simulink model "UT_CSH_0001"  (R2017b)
settings: Solver=FixedStepDiscrete  StartTime=0.0  StopTime=2  FixedStep=0.01  RelTol=1e-3  EnableMultiTasking=on
undefined symbols (not defined in the file): sigbuilder_block

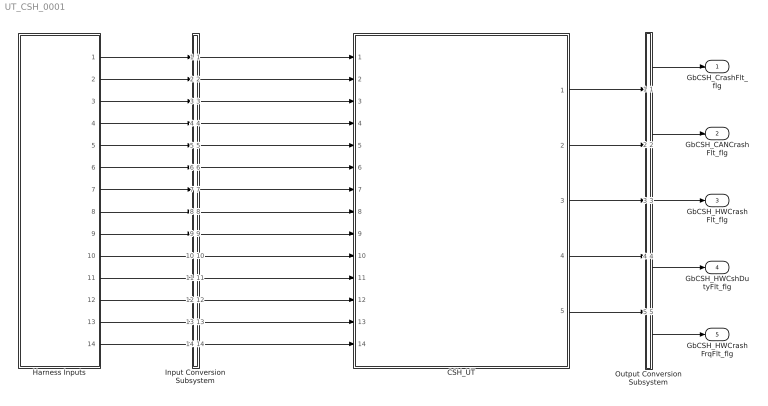
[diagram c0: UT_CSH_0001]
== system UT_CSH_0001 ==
  CSH_UT : ModelReference  ModelNameDialog=CSH_UT  SimulationMode=Normal  ModelReferenceVersion='M102C102'
  Harness Inputs : Subsystem  Tag=STV Subsys  LoadFcn=sigbuilder_block('load');  StartFcn=sigbuilder_block('start');  StopFcn=sigbuilder_block('stop');  ClipboardFcn=sigbuilder_block('clipboard');  mask(Sigbuilder block){tuvar=[0:10]}
      mask init:
      | if ~strcmp(get_param(bdroot(gcb),'SimulationStatus'),'stopped'),tuvar = sigbuilder_block('maskInit'); end
  Input Conversion Subsystem : Subsystem  Tag=__SLT_ICS__  Description=Signal spec. and routing
  Output Conversion Subsystem : Subsystem  Tag=__SLT_OCS__  Description=Signal spec. and routing
  GbCSH_CrashFlt_flg : Outport  OutDataTypeStr=boolean  PortDimensions=[1]
  GbCSH_CANCrashFlt_flg : Outport  Port=2  OutDataTypeStr=boolean  PortDimensions=[1]
  GbCSH_HWCrashFlt_flg : Outport  Port=3  OutDataTypeStr=boolean  PortDimensions=[1]
  GbCSH_HWCshDutyFlt_flg : Outport  Port=4  OutDataTypeStr=boolean  PortDimensions=[1]
  GbCSH_HWCrashFrqFlt_flg : Outport  Port=5  OutDataTypeStr=boolean  PortDimensions=[1]
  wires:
  Harness Inputs/1(GeADP_CrashSgl_enum) -> Input Conversion Subsystem/1(Inport_1)
  Harness Inputs/2(GcLDP_CshDutyOut_pct) -> Input Conversion Subsystem/2(Inport_2)
  Harness Inputs/3(GcLDP_CshPerOut_ms) -> Input Conversion Subsystem/3(Inport_3)
  Harness Inputs/4(GcLDP_CshSt_numb) -> Input Conversion Subsystem/4(Inport_4)
  Harness Inputs/5(GcLDP_CshDutyFbk_pct) -> Input Conversion Subsystem/5(Inport_5)
  Harness Inputs/6(GcLDP_CshPerFbk_ms) -> Input Conversion Subsystem/6(Inport_6)
  Harness Inputs/7(GcLDP_CshStFbk_numb) -> Input Conversion Subsystem/7(Inport_7)
  Harness Inputs/8(GbWSM_Kl15WkUpPrs_flg) -> Input Conversion Subsystem/8(Inport_8)
  Harness Inputs/9(GbUDS_TestMode1_flg) -> Input Conversion Subsystem/9(Inport_9)
  Harness Inputs/10(GeUDS_PrjSel_enum) -> Input Conversion Subsystem/10(Inport_10)
  Harness Inputs/11(GbADP_050ChkSum_flg) -> Input Conversion Subsystem/11(Inport_11)
  Harness Inputs/12(GbADP_050RCMsg_flg) -> Input Conversion Subsystem/12(Inport_12)
  Harness Inputs/13(GbISP_TF050ChkSum_flg) -> Input Conversion Subsystem/13(Inport_13)
  Harness Inputs/14(GbISP_TF050RCMsg_flg) -> Input Conversion Subsystem/14(Inport_14)
  Output Conversion Subsystem/1(Outport_1) -> GbCSH_CrashFlt_flg/1
  Output Conversion Subsystem/2(Outport_2) -> GbCSH_CANCrashFlt_flg/1
  Output Conversion Subsystem/3(Outport_3) -> GbCSH_HWCrashFlt_flg/1
  Output Conversion Subsystem/4(Outport_4) -> GbCSH_HWCshDutyFlt_flg/1
  Output Conversion Subsystem/5(Outport_5) -> GbCSH_HWCrashFrqFlt_flg/1
  Input Conversion Subsystem/1(Outport_1) -> CSH_UT/1
  Input Conversion Subsystem/2(Outport_2) -> CSH_UT/2
  Input Conversion Subsystem/3(Outport_3) -> CSH_UT/3
  Input Conversion Subsystem/4(Outport_4) -> CSH_UT/4
  Input Conversion Subsystem/5(Outport_5) -> CSH_UT/5
  Input Conversion Subsystem/6(Outport_6) -> CSH_UT/6
  Input Conversion Subsystem/7(Outport_7) -> CSH_UT/7
  Input Conversion Subsystem/8(Outport_8) -> CSH_UT/8
  Input Conversion Subsystem/9(Outport_9) -> CSH_UT/9
  Input Conversion Subsystem/10(Outport_10) -> CSH_UT/10
  Input Conversion Subsystem/11(Outport_11) -> CSH_UT/11
  Input Conversion Subsystem/12(Outport_12) -> CSH_UT/12
  Input Conversion Subsystem/13(Outport_13) -> CSH_UT/13
  Input Conversion Subsystem/14(Outport_14) -> CSH_UT/14
  CSH_UT/1 -> Output Conversion Subsystem/1(Inport_1)
  CSH_UT/2 -> Output Conversion Subsystem/2(Inport_2)
  CSH_UT/3 -> Output Conversion Subsystem/3(Inport_3)
  CSH_UT/4 -> Output Conversion Subsystem/4(Inport_4)
  CSH_UT/5 -> Output Conversion Subsystem/5(Inport_5)

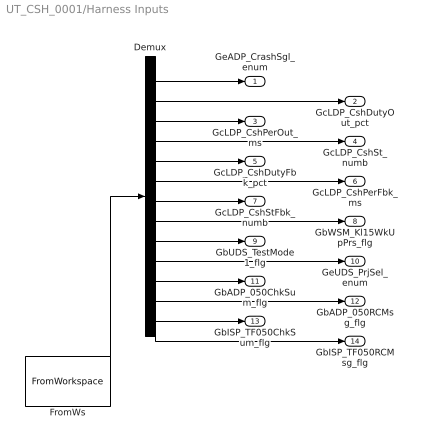
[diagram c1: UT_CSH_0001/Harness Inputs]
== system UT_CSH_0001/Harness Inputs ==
  Demux : Demux  Tag=STV Demux  Outputs=14
  FromWs : FromWorkspace  Tag=STV FromWs  VariableName=tuvar  SampleTime=0
  GeADP_CrashSgl_enum : Outport  Tag=STV Outport
  GcLDP_CshDutyOut_pct : Outport  Tag=STV Outport  Port=2
  GcLDP_CshPerOut_ms : Outport  Tag=STV Outport  Port=3
  GcLDP_CshSt_numb : Outport  Tag=STV Outport  Port=4
  GcLDP_CshDutyFbk_pct : Outport  Tag=STV Outport  Port=5
  GcLDP_CshPerFbk_ms : Outport  Tag=STV Outport  Port=6
  GcLDP_CshStFbk_numb : Outport  Tag=STV Outport  Port=7
  GbWSM_Kl15WkUpPrs_flg : Outport  Tag=STV Outport  Port=8
  GbUDS_TestMode1_flg : Outport  Tag=STV Outport  Port=9
  GeUDS_PrjSel_enum : Outport  Tag=STV Outport  Port=10
  GbADP_050ChkSum_flg : Outport  Tag=STV Outport  Port=11
  GbADP_050RCMsg_flg : Outport  Tag=STV Outport  Port=12
  GbISP_TF050ChkSum_flg : Outport  Tag=STV Outport  Port=13
  GbISP_TF050RCMsg_flg : Outport  Tag=STV Outport  Port=14
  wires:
  FromWs/1 -> Demux/1
  Demux/1 -> GeADP_CrashSgl_enum/1
  Demux/2 -> GcLDP_CshDutyOut_pct/1
  Demux/3 -> GcLDP_CshPerOut_ms/1
  Demux/4 -> GcLDP_CshSt_numb/1
  Demux/5 -> GcLDP_CshDutyFbk_pct/1
  Demux/6 -> GcLDP_CshPerFbk_ms/1
  Demux/7 -> GcLDP_CshStFbk_numb/1
  Demux/8 -> GbWSM_Kl15WkUpPrs_flg/1
  Demux/9 -> GbUDS_TestMode1_flg/1
  Demux/10 -> GeUDS_PrjSel_enum/1
  Demux/11 -> GbADP_050ChkSum_flg/1
  Demux/12 -> GbADP_050RCMsg_flg/1
  Demux/13 -> GbISP_TF050ChkSum_flg/1
  Demux/14 -> GbISP_TF050RCMsg_flg/1

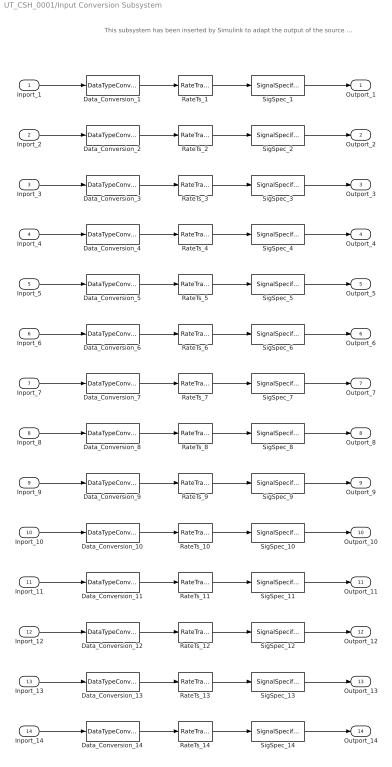
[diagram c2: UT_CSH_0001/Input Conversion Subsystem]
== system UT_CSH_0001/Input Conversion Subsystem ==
  note: This subsystem has been inserted by Simulink to adapt the output of the source blocks to the interface required by the harnessed component. Modifying the contents of this subsystem may result in compilation and simulation failure.
  Inport_1 : Inport
  Inport_2 : Inport  Port=2
  Inport_3 : Inport  Port=3
  Inport_4 : Inport  Port=4
  Inport_5 : Inport  Port=5
  Inport_6 : Inport  Port=6
  Inport_7 : Inport  Port=7
  Inport_8 : Inport  Port=8
  Inport_9 : Inport  Port=9
  Inport_10 : Inport  Port=10
  Inport_11 : Inport  Port=11
  Inport_12 : Inport  Port=12
  Inport_13 : Inport  Port=13
  Inport_14 : Inport  Port=14
  Data_Conversion_{1..2,4..5,7,10} (6 alike) : DataTypeConversion  OutDataTypeStr=uint8
  Data_Conversion_{8..9,11..14} (6 alike) : DataTypeConversion  OutDataTypeStr=boolean
  Data_Conversion_3 : DataTypeConversion  OutDataTypeStr=uint32
  Data_Conversion_6 : DataTypeConversion  OutDataTypeStr=uint32
  RateTs_{1..14} (14 alike) : RateTransition  OutPortSampleTime=0.01
  SigSpec_1 : SignalSpecification  OutDataTypeStr=uint8  Unit=enum  Dimensions=[1]  SampleTime=0.01
  SigSpec_10 : SignalSpecification  OutDataTypeStr=uint8  Unit=numb  Dimensions=[1]  SampleTime=0.01
  SigSpec_11 : SignalSpecification  OutDataTypeStr=boolean  Unit=flg  Dimensions=[1]  SampleTime=0.01
  SigSpec_12 : SignalSpecification  OutDataTypeStr=boolean  Unit=flg  Dimensions=[1]  SampleTime=0.01
  SigSpec_13 : SignalSpecification  OutDataTypeStr=boolean  Unit=flag  Dimensions=[1]  SampleTime=0.01
  SigSpec_14 : SignalSpecification  OutDataTypeStr=boolean  Unit=flag  Dimensions=[1]  SampleTime=0.01
  SigSpec_2 : SignalSpecification  OutDataTypeStr=uint8  Unit=%  Dimensions=[1]  SampleTime=0.01
  SigSpec_3 : SignalSpecification  OutDataTypeStr=uint32  Unit=ms  Dimensions=[1]  SampleTime=0.01
  SigSpec_4 : SignalSpecification  OutDataTypeStr=uint8  Unit=NA  Dimensions=[1]  SampleTime=0.01
  SigSpec_5 : SignalSpecification  OutDataTypeStr=uint8  Unit=%  Dimensions=[1]  SampleTime=0.01
  SigSpec_6 : SignalSpecification  OutDataTypeStr=uint32  Unit=ms  Dimensions=[1]  SampleTime=0.01
  SigSpec_7 : SignalSpecification  OutDataTypeStr=uint8  Unit=numb  Dimensions=[1]  SampleTime=0.01
  SigSpec_8 : SignalSpecification  OutDataTypeStr=boolean  Unit=flg  Dimensions=[1]  SampleTime=0.01
  SigSpec_9 : SignalSpecification  OutDataTypeStr=boolean  Unit=flag  Dimensions=[1]  SampleTime=0.01
  Outport_1 : Outport
  Outport_2 : Outport  Port=2
  Outport_3 : Outport  Port=3
  Outport_4 : Outport  Port=4
  Outport_5 : Outport  Port=5
  Outport_6 : Outport  Port=6
  Outport_7 : Outport  Port=7
  Outport_8 : Outport  Port=8
  Outport_9 : Outport  Port=9
  Outport_10 : Outport  Port=10
  Outport_11 : Outport  Port=11
  Outport_12 : Outport  Port=12
  Outport_13 : Outport  Port=13
  Outport_14 : Outport  Port=14
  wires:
  SigSpec_1/1 -> Outport_1/1
  RateTs_1/1 -> SigSpec_1/1
  Data_Conversion_1/1 -> RateTs_1/1
  Inport_1/1 -> Data_Conversion_1/1
  SigSpec_2/1 -> Outport_2/1
  RateTs_2/1 -> SigSpec_2/1
  Data_Conversion_2/1 -> RateTs_2/1
  Inport_2/1 -> Data_Conversion_2/1
  SigSpec_3/1 -> Outport_3/1
  RateTs_3/1 -> SigSpec_3/1
  Data_Conversion_3/1 -> RateTs_3/1
  Inport_3/1 -> Data_Conversion_3/1
  SigSpec_4/1 -> Outport_4/1
  RateTs_4/1 -> SigSpec_4/1
  Data_Conversion_4/1 -> RateTs_4/1
  Inport_4/1 -> Data_Conversion_4/1
  SigSpec_5/1 -> Outport_5/1
  RateTs_5/1 -> SigSpec_5/1
  Data_Conversion_5/1 -> RateTs_5/1
  Inport_5/1 -> Data_Conversion_5/1
  SigSpec_6/1 -> Outport_6/1
  RateTs_6/1 -> SigSpec_6/1
  Data_Conversion_6/1 -> RateTs_6/1
  Inport_6/1 -> Data_Conversion_6/1
  SigSpec_7/1 -> Outport_7/1
  RateTs_7/1 -> SigSpec_7/1
  Data_Conversion_7/1 -> RateTs_7/1
  Inport_7/1 -> Data_Conversion_7/1
  SigSpec_8/1 -> Outport_8/1
  RateTs_8/1 -> SigSpec_8/1
  Data_Conversion_8/1 -> RateTs_8/1
  Inport_8/1 -> Data_Conversion_8/1
  SigSpec_9/1 -> Outport_9/1
  RateTs_9/1 -> SigSpec_9/1
  Data_Conversion_9/1 -> RateTs_9/1
  Inport_9/1 -> Data_Conversion_9/1
  SigSpec_10/1 -> Outport_10/1
  RateTs_10/1 -> SigSpec_10/1
  Data_Conversion_10/1 -> RateTs_10/1
  Inport_10/1 -> Data_Conversion_10/1
  SigSpec_11/1 -> Outport_11/1
  RateTs_11/1 -> SigSpec_11/1
  Data_Conversion_11/1 -> RateTs_11/1
  Inport_11/1 -> Data_Conversion_11/1
  SigSpec_12/1 -> Outport_12/1
  RateTs_12/1 -> SigSpec_12/1
  Data_Conversion_12/1 -> RateTs_12/1
  Inport_12/1 -> Data_Conversion_12/1
  SigSpec_13/1 -> Outport_13/1
  RateTs_13/1 -> SigSpec_13/1
  Data_Conversion_13/1 -> RateTs_13/1
  Inport_13/1 -> Data_Conversion_13/1
  SigSpec_14/1 -> Outport_14/1
  RateTs_14/1 -> SigSpec_14/1
  Data_Conversion_14/1 -> RateTs_14/1
  Inport_14/1 -> Data_Conversion_14/1

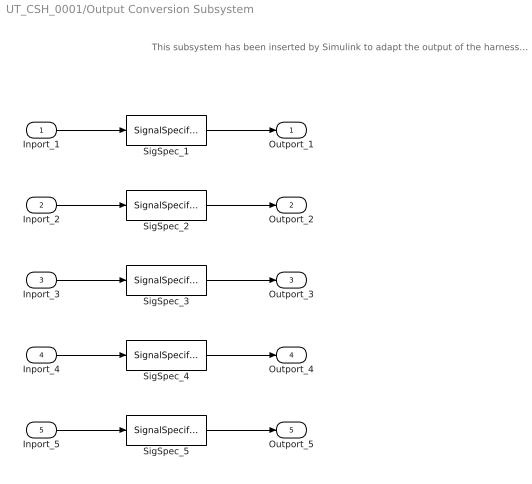
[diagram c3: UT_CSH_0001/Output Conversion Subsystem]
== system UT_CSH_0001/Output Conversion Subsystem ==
  note: This subsystem has been inserted by Simulink to adapt the output of the harnessed component to the interface required by the sink blocks. Modifying the contents of this subsystem may result in compilation and simulation failure.
  Inport_1 : Inport
  Inport_2 : Inport  Port=2
  Inport_3 : Inport  Port=3
  Inport_4 : Inport  Port=4
  Inport_5 : Inport  Port=5
  SigSpec_1 : SignalSpecification  OutDataTypeStr=boolean  Unit=flag  Dimensions=[1]
  SigSpec_{2..5} (4 alike) : SignalSpecification  OutDataTypeStr=boolean  Unit=flag  Dimensions=[1]  SampleTime=0.01
  Outport_1 : Outport
  Outport_2 : Outport  Port=2
  Outport_3 : Outport  Port=3
  Outport_4 : Outport  Port=4
  Outport_5 : Outport  Port=5
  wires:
  Inport_1/1 -> SigSpec_1/1
  SigSpec_1/1 -> Outport_1/1
  Inport_2/1 -> SigSpec_2/1
  SigSpec_2/1 -> Outport_2/1
  Inport_3/1 -> SigSpec_3/1
  SigSpec_3/1 -> Outport_3/1
  Inport_4/1 -> SigSpec_4/1
  SigSpec_4/1 -> Outport_4/1
  Inport_5/1 -> SigSpec_5/1
  SigSpec_5/1 -> Outport_5/1
